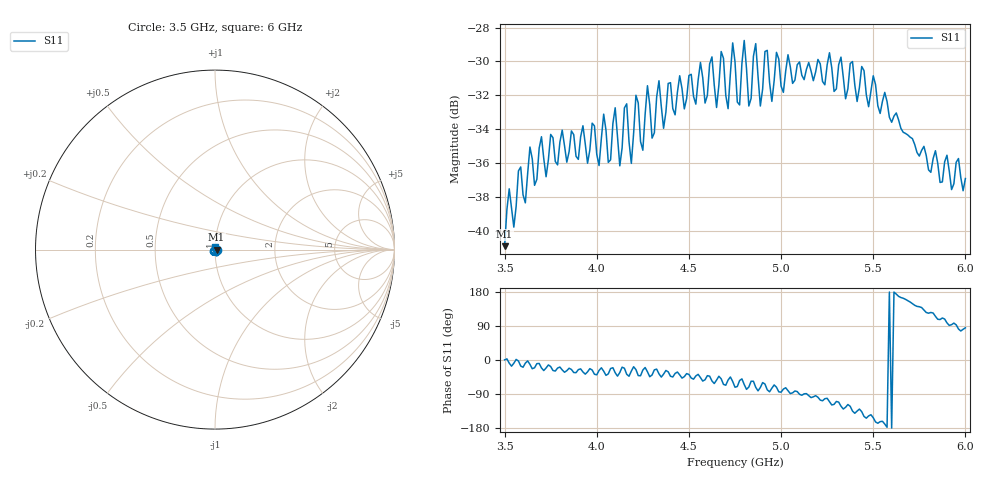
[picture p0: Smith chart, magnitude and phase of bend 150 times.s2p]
!  31/07/2025  12:57:43
! Ref Plane: 0.000 mm
# MHZ S MA R  50
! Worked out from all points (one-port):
!   201 points, 3.5 GHz to 6 GHz, reference 50 ohm
!   lowest |S11| = -40.9 dB at 3.5 GHz (marker M1), VSWR 1.02, Z = 50.9 + j0.00722 ohm
!   |S11| at or under -10 dB: start of sweep to end of sweep
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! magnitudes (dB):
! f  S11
! 3.5 GHz  -40.9
! 3.638 GHz  -35.0
! 3.812 GHz  -34.0
! 4.013 GHz  -36.1
! 4.037 GHz  -33.1
! 4.062 GHz  -36.0
! 4.1 GHz  -32.7
! 4.125 GHz  -36.2
! 4.162 GHz  -32.5
! 4.188 GHz  -36.0
! 4.213 GHz  -32.0
! 4.25 GHz  -35.2
! 4.275 GHz  -31.4
! 4.3 GHz  -34.5
! 4.338 GHz  -31.1
! 4.362 GHz  -33.9
! 4.438 GHz  -31.8
! 4.625 GHz  -29.7
! 4.65 GHz  -32.7
! 4.675 GHz  -29.4
! 4.713 GHz  -32.8
! 4.75 GHz  -30.0
! 4.775 GHz  -32.6
! 4.8 GHz  -28.8
! 5.062 GHz  -31.3
! 5.375 GHz  -30.1
! 5.688 GHz  -34.3
! 6 GHz  -36.9
